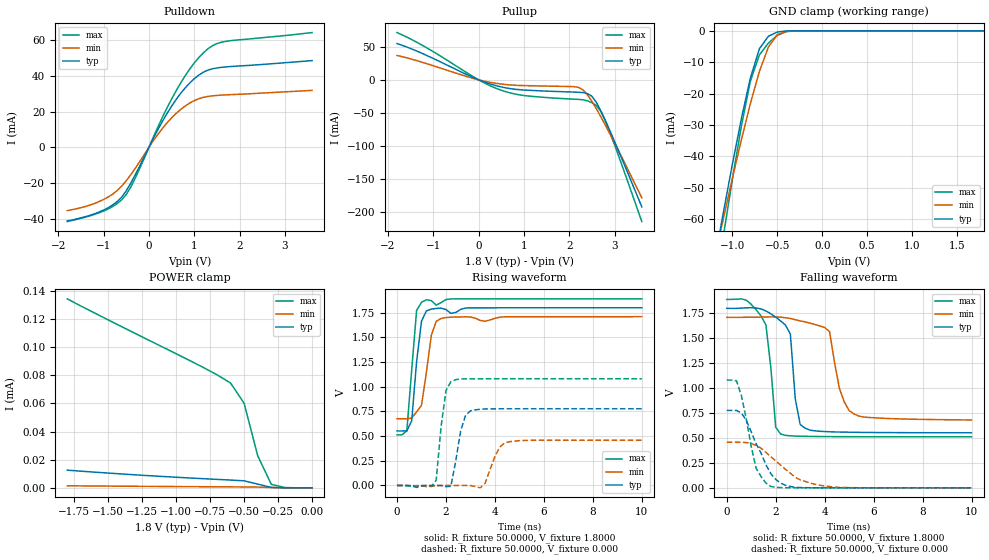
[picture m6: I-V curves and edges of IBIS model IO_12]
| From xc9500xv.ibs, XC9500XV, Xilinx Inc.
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|   Model IO_12
[Model]   IO_12
Model_type   I/O
Polarity   Non-Inverting
Enable   Active-High
Vinl =   0.8000V
Vinh =   2.0000V
Vmeas =   0.8000V
Cref =  35.0000pF
Rref =   1.0000M
Vref =  0.000V
C_comp   1.8820pF   1.2910pF   2.4730pF
[Temperature Range]   25.0000   100.0000   0.000
[Voltage Range]   1.8000V   1.7100V   1.8900V
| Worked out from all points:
|   slope of the pulldown table from 0 to 0.27 V, typ, clamps not added: 20.4 ohm
|   slope of the pullup table from 0 to 0.27 V, typ, clamps not added: 40.8 ohm
|   GND clamp passes 1 mA (typ) near -0.55 V on its own axis
|   rising waveform, R_fixture 50.0000, V_fixture 1.8000: 20-80 % time 296ps typ, 349ps min, 271ps max; typ from 0.552 V to 1.8 V
|   rising waveform, R_fixture 50.0000, V_fixture 0.000: 20-80 % time 359ps typ, 453ps min, 287ps max; typ from 0 V to 0.776 V
|   falling waveform, R_fixture 50.0000, V_fixture 1.8000: 20-80 % time 290ps typ, 523ps min, 331ps max; typ from 1.8 V to 0.552 V
|   falling waveform, R_fixture 50.0000, V_fixture 0.000: 20-80 % time 876ps typ, 1.36ns min, 532ps max; typ from 0.776 V to 0 V
[Pulldown]
| voltage   I(typ)   I(min)   I(max)
-1.8V     -40.9mA    -35.2mA    -41.3mA
-1.3V     -37.85mA   -32.1mA    -38.1mA
-900mV    -33.61mA   -27.65mA   -34.3mA
-700mV    -30.16mA   -24.04mA   -31.27mA
-500mV    -24.2mA    -18.6mA    -26.23mA
-300mV    -15.14mA   -11.58mA   -16.99mA
200mV     10.04mA    7.385mA    11.51mA
500mV     22.99mA    16.49mA    26.96mA
900mV     35.93mA    24.75mA    43.66mA
1.3V      43.1mA     28.44mA    54.96mA
1.7V      44.91mA    29.32mA    59.17mA
3.6V      48.42mA    31.83mA    64.04mA
[Pullup]
| voltage   I(typ)   I(min)   I(max)
-1.8V     54.98mA    36.8mA     71.63mA
-1.2V     38.67mA    25.69mA    50.7mA
-100mV    2.906mA    1.804mA    4.051mA
400mV     -9.157mA   -5.475mA   -13.28mA
1V        -15.43mA   -8.73mA    -23.81mA
2.2V      -18.82mA   -11.34mA   -29.66mA
2.4V      -20.89mA   -22.62mA   -31.86mA
2.5V      -25.06mA   -32.71mA   -34.73mA
2.6V      -34.53mA   -44.2mA    -38.98mA
2.7V      -47.58mA   -56.51mA   -48.25mA
2.9V      -77.68mA   -82.5mA    -80.44mA
3.6V      -192.6mA   -178.9mA   -214.9mA
[GND_clamp]
| voltage   I(typ)   I(min)   I(max)
-1.8V     -171.6mA   -154.7mA   -199.4mA
-1.2V     -73.41mA   -72.77mA   -83.79mA
-1.1V     -57.66mA   -59.67mA   -65.18mA
-1V       -42.38mA   -46.9mA    -47.16mA
-900mV    -27.9mA    -34.63mA   -30.27mA
-800mV    -15.03mA   -23.14mA   -16.01mA
-700mV    -5.733mA   -12.98mA   -7.683mA
-600mV    -1.741mA   -5.183mA   -3.919mA
-500mV    -371uA     -1.195mA   -1.434mA
-400mV    -43.13uA   -156.2uA   -255.7uA
-200mV    -89.07nA   -475.8nA   -857.8nA
1.8V      335pA      7.049nA    1.584nA
[POWER_clamp]
| voltage   I(typ)   I(min)   I(max)
-1.8V     12.57uA    1.465uA    134.3uA
-800mV    6.509uA    806.2nA    85.56uA
-600mV    5.532uA    702nA      74.53uA
-500mV    4.994uA    650.2nA    60.11uA
-400mV    2.651uA    538.7nA    22.85uA
-300mV    324.7nA    232.1nA    2.491uA
-200mV    23.09nA    31.76nA    201.3nA
0V        335.2pA    3.931nA    2.176nA
[Ramp]
| variable   typ   min   max
dV/dt_r   0.4658/0.3199n   0.2745/0.4532n   0.6486/0.2427n
dV/dt_f   0.7487/0.2770n   0.6175/0.3952n   0.8266/0.2581n
R_load = 50.0000
[Rising Waveform]
R_fixture = 50.0000
V_fixture = 1.8000
V_fixture_min = 1.7100
V_fixture_max = 1.8900
L_fixture = 0.000H
C_fixture = 0.000F
| time   V(typ)   V(min)   V(max)
0s        551.9mV    676mV      512.4mV
400ps     552.4mV    675.8mV    552.9mV
600ps     655.4mV    681.7mV    1.173V
800ps     1.254V     746.4mV    1.773V
1ns       1.664V     812.7mV    1.855V
1.4ns     1.786V     1.52V      1.873V
1.6ns     1.793V     1.662V     1.827V
1.8ns     1.796V     1.692V     1.852V
2.2ns     1.742V     1.704V     1.889V
10ns      1.8V       1.71V      1.89V
[Rising Waveform]
R_fixture = 50.0000
V_fixture = 0.000
V_fixture_min = 0.000
V_fixture_max = 0.000
L_fixture = 0.000H
C_fixture = 0.000F
| time   V(typ)   V(min)   V(max)
0s        0V         0V         0V
1.6ns     -86.69uV   -1.73mV    52.67mV
1.8ns     -51.86uV   -660.9uV   596.3mV
2ns       -11.86mV   -290.5uV   960.6mV
2.2ns     -9.18mV    -112.2uV   1.052V
2.6ns     553.9mV    25.45uV    1.079V
3ns       755.2mV    -1.159mV   1.08V
3.6ns     774.8mV    22.87mV    1.081V
4.4ns     776.4mV    431mV      1.081V
10ns      776.3mV    457.5mV    1.081V
[Falling Waveform]
R_fixture = 50.0000
V_fixture = 1.8000
V_fixture_min = 1.7100
V_fixture_max = 1.8900
L_fixture = 0.000H
C_fixture = 0.000F
| time   V(typ)   V(min)   V(max)
0s        1.8V       1.71V      1.89V
1.6ns     1.774V     1.714V     1.635V
2ns       1.712V     1.714V     608mV
2.2ns     1.674V     1.712V     540.2mV
2.6ns     1.542V     1.698V     521.7mV
2.8ns     894.1mV    1.686V     519mV
3.2ns     598.7mV    1.665V     516.7mV
4.2ns     562.5mV    1.567V     513.9mV
5.2ns     557.3mV    740.5mV    513.1mV
10ns      552.2mV    680.9mV    512.4mV
[Falling Waveform]
R_fixture = 50.0000
V_fixture = 0.000
V_fixture_min = 0.000
V_fixture_max = 0.000
L_fixture = 0.000H
C_fixture = 0.000F
| time   V(typ)   V(min)   V(max)
0s        776.3mV    457mV      1.081V
400ps     776.1mV    457mV      1.073V
600ps     750.5mV    456.6mV    924mV
800ps     675.7mV    454.1mV    688.6mV
1.2ns     441.9mV    425.7mV    196.8mV
1.8ns     142.7mV    313.2mV    14.14mV
2.4ns     25.86mV    185.8mV    1.194mV
3ns       2.821mV    80.01mV    374.8uV
3.8ns     618.3uV    26.27mV    155.6uV
10ns      32.75uV    139.1uV    1.688uV
